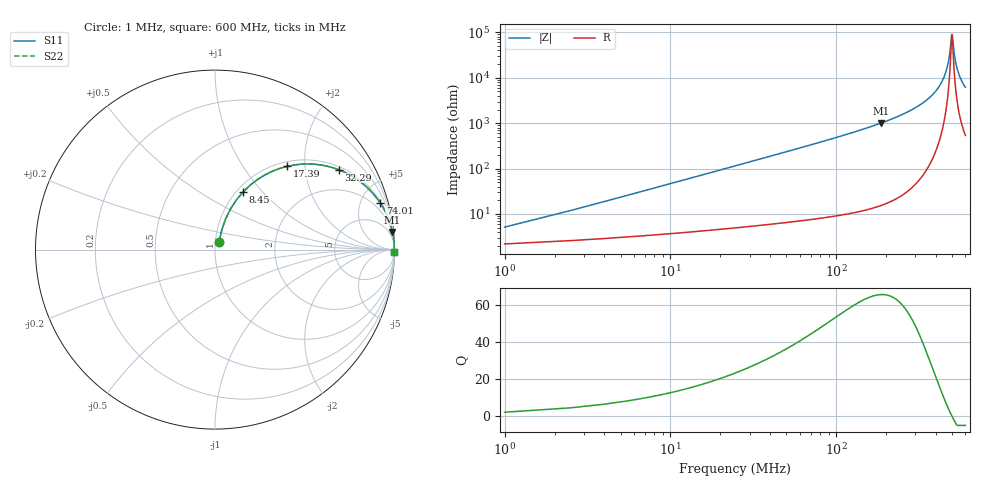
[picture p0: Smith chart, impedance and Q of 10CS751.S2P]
! Coilcraft 1008CS-751 Chip Inductor
! 02 July 2002
# MHZ S MA R 50
!Freq  MagS11  AngS11  MagS21  AngS21  MagS12  AngS12  MagS22  AngS22
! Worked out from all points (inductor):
!   404 points, 1 MHz to 600 MHz, reference 50 ohm
!   read as one part in series: L = 740 nH near 3.98 MHz
!   highest Q = 65.4 at 185.8 MHz (marker M1), where L = 860 nH
!   self-resonance near 497.2 MHz
!   S11 on the Smith chart (normalised r, x): 1 MHz: 1.04, +0.09; 8.45 MHz: 1.07, +0.79; 17.39 MHz: 1.09, +1.62; 32.29 MHz: 1.11, +3.02; 74.01 MHz: 1.15, +7.04; 600 MHz: open
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1  0.05024 62.2  0.9776 -2.6  0.9776 -2.6  0.05024 62.2
5.47  0.2413 69.2  0.9416 -13.9  0.9416 -13.9  0.2413 69.2
8.45  0.3564 64.1  0.9032 -20.8  0.9032 -20.8  0.3564 64.1
12.92  0.5016 56.2  0.8326 -30.0  0.8326 -30.0  0.5016 56.2
17.39  0.6137 49.1  0.757 -37.8  0.757 -37.8  0.6137 49.1
32.29  0.82 32.9  0.5435 -55.0  0.5435 -55.0  0.82 32.9
48.68  0.9069 23.4  0.3967 -65.0  0.3967 -65.0  0.9069 23.4
74.01  0.9564 15.8  0.2717 -73.0  0.2717 -73.0  0.9564 15.8
102.32  0.9768 11.3  0.1966 -77.6  0.1966 -77.6  0.9768 11.3
185.76  0.9936 5.7  0.09903 -83.4  0.09903 -83.4  0.9936 5.7
202.15  0.9947 5.1  0.08839 -84.0  0.08839 -84.0  0.9947 5.1
301.98  0.9981 2.6  0.04496 -86.2  0.04496 -86.2  0.9981 2.6
401.81  0.9989 1.1  0.01869 -86.1  0.01869 -86.1  0.9989 1.1
434.59  0.999 0.7  0.01184 -84.6  0.01184 -84.6  0.999 0.7
459.92  0.999 0.4  0.006963 -81.2  0.006963 -81.2  0.999 0.4
479.29  0.9989 0.2  0.003489 -72.1  0.003489 -72.1  0.9989 0.2
495.68  0.9989 0.0  0.001179 -21.0  0.001179 -21.0  0.9989 0.0
501.64  0.9989 -0.0  0.00127 28.5  0.00127 28.5  0.9989 -0.0
516.54  0.9988 -0.2  0.003337 69.6  0.003337 69.6  0.9988 -0.2
534.42  0.9988 -0.3  0.006187 78.5  0.006187 78.5  0.9988 -0.3
561.24  0.9987 -0.6  0.01039 82.3  0.01039 82.3  0.9987 -0.6
600  0.9985 -0.9  0.01619 84.1  0.01619 84.1  0.9985 -0.9
